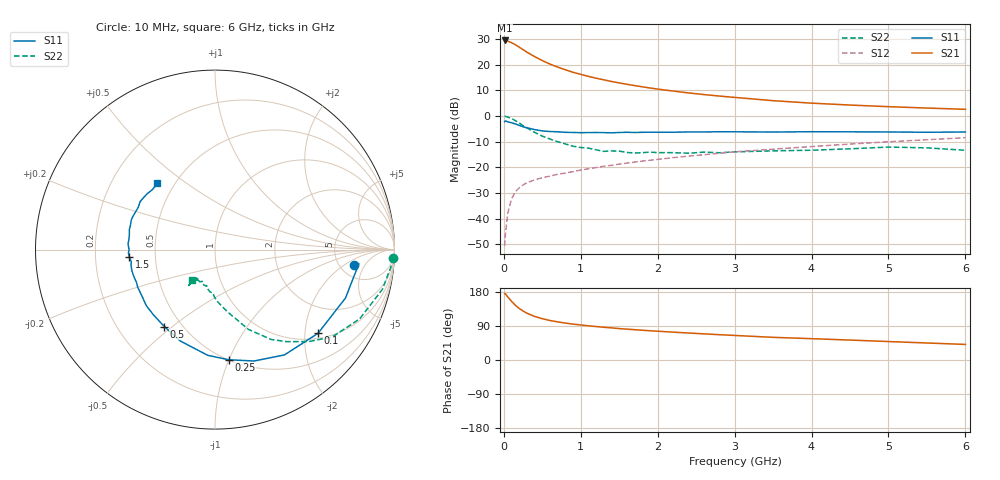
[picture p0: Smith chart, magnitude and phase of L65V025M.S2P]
!  INFINEON TECHNOLOGIES Small Signal Semiconductors
! BFR380L3 , Si-NPN RF-Transistor in TSLP-3-1
!  Vce=5 V,  Ic=25 mA
! Common Emitter S-Parameters:  07. March 2005
#  GHz  S  MA  R  50
! f  S11  S21  S12  S22
! GHz  Mag  Ang  Mag  Ang  Mag  Ang  Mag  Ang
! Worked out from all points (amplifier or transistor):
!   36 points, 10 MHz to 6 GHz, reference 50 ohm
!   highest |S21| = 29.5 dB at 10 MHz (marker M1)
!   |S21| within 3 dB of that: start of sweep to 219.4 MHz
!   unconditionally stable (mu >= 1): 2.204 GHz to 4.761 GHz
!   at 250 MHz: K = 0.33, MSG = 26.4 dB, |S12| = -26.9 dB
!   at 1.4 GHz: K = 0.93, MSG = 16.3 dB, |S12| = -19.2 dB
!   at 6 GHz: K = 0.97, MSG = 5.5 dB, |S12| = -8.5 dB
!   S11 on the Smith chart (normalised r, x): 10 MHz: 6.65, -2.96; 100 MHz: 1.14, -2.34; 250 MHz: 0.50, -1.00; 500 MHz: 0.40, -0.47; 1.5 GHz: 0.35, -0.04; 6 GHz: 0.40, +0.39
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0.01  0.7777 -6.5  29.85 175.3  0.0029 80.4  0.9955 -2.6
0.02  0.8058 -5.6  29.62 174.7  0.0049 82.9  0.9853 -5.5
0.05  0.7753 -20.4  28.99 166.7  0.0125 82.3  0.959 -13.3
0.1  0.7396 -39.1  26.98 154.9  0.0242 72.4  0.8935 -25.6
0.15  0.7029 -56.6  24.64 144.4  0.0335 65.4  0.8153 -36.6
0.2  0.6577 -70.7  22.06 136.0  0.0398 60.8  0.7323 -44.4
0.25  0.6184 -82.9  19.75 129.3  0.0453 56.5  0.6509 -52.0
0.3  0.5906 -93.9  17.66 123.5  0.0502 54.9  0.5906 -58.0
0.4  0.5447 -110.8  14.46 115.0  0.0569 51.7  0.4808 -67.4
0.5  0.5133 -123.4  12.1 109.0  0.0627 52.0  0.4072 -72.8
0.6  0.4998 -133.4  10.32 104.2  0.0675 51.9  0.3564 -78.4
0.7  0.4938 -140.8  9.022 100.6  0.0733 53.2  0.3158 -83.3
0.9  0.4788 -154.0  7.15 94.7  0.0826 55.2  0.2584 -91.4
1.1  0.4767 -162.0  5.946 90.2  0.0938 56.7  0.2366 -97.1
1.5  0.4785 -174.8  4.434 82.9  0.1155 59.6  0.2073 -107.1
1.8  0.4826 177.8  3.725 78.5  0.1324 60.8  0.193 -112.5
2.2  0.484 170.4  3.076 73.5  0.1545 61.8  0.1933 -116.8
2.8  0.4948 160.5  2.458 66.8  0.188 62.7  0.1925 -124.6
3.5  0.4884 151.1  1.997 59.8  0.2263 61.5  0.2098 -125.2
4.5  0.493 144.8  1.64 52.6  0.2845 60.9  0.2298 -125.9
5.5  0.483 136.3  1.433 44.9  0.3458 58.0  0.2399 -126.1
6  0.4895 130.9  1.355 41.1  0.378 56.1  0.2152 -127.2
